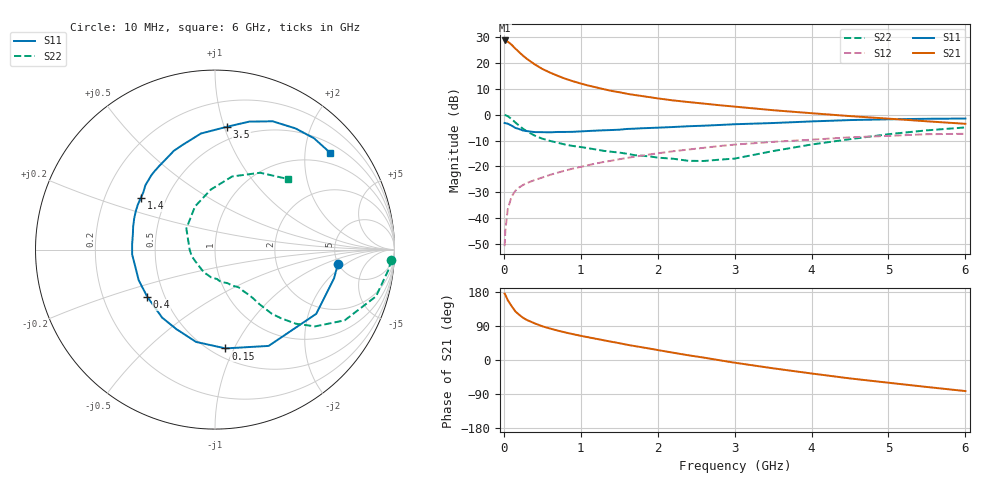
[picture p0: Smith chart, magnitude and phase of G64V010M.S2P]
! SIEMENS Small Signal Semiconductors
! BFG193
! Si NPN RF Bipolar Junction Transistor in SOT223
! VCE = 4 V  IC = 10 mA
! Common Emitter S-Parameters:  August  1996
# GHz  S  MA  R  50
!  f  S11  S21  S12  S22
! GHz  MAG  ANG  MAG  ANG  MAG  ANG  MAG  ANG
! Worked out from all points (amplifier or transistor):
!   36 points, 10 MHz to 6 GHz, reference 50 ohm
!   highest |S21| = 28.6 dB at 10 MHz (marker M1)
!   |S21| within 3 dB of that: start of sweep to 145.5 MHz
!   unconditionally stable (mu >= 1): 884.1 MHz to 2.514 GHz
!   at 250 MHz: K = 0.54, MSG = 24.9 dB, |S12| = -27.2 dB
!   at 1.4 GHz: K = 1.07, MAG = 11.9 dB, |S12| = -17.8 dB
!   at 6 GHz: K = 0.87, MSG = 1.9 dB, |S12| = -7.4 dB
!   S11 on the Smith chart (normalised r, x): 10 MHz: 4.93, -1.53; 150 MHz: 0.58, -0.92; 400 MHz: 0.40, -0.27; 1.4 GHz: 0.36, +0.28; 3.5 GHz: 0.39, +1.02; 6 GHz: 0.71, +2.58
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0.01  0.6889 -6.8  26.88 175.2  0.0029 89.8  0.9842 -3.3
0.02  0.6825 -13.5  26.8 171.8  0.0058 86.3  0.9729 -6.7
0.05  0.6679 -32.4  25.57 158.4  0.0147 75.8  0.9341 -16.2
0.1  0.6142 -60.9  22.3 142.5  0.0262 65.7  0.8232 -28.6
0.15  0.5535 -84.0  18.73 128.3  0.034 57.4  0.7028 -37.5
0.2  0.525 -101.6  15.95 119.2  0.0394 54.1  0.6112 -42.5
0.25  0.4927 -115.8  13.64 111.4  0.0439 51.3  0.5313 -46.1
0.3  0.48 -127.9  11.87 105.5  0.0479 50.8  0.4764 -48.5
0.4  0.4599 -145.1  9.327 96.8  0.0546 50.4  0.3938 -50.8
0.5  0.4581 -158.2  7.597 89.0  0.0611 49.9  0.3434 -52.0
0.6  0.4542 -167.9  6.457 83.1  0.0688 50.5  0.3112 -53.4
0.7  0.4624 -176.6  5.591 77.6  0.0759 51.3  0.286 -55.2
0.9  0.4655 169.4  4.388 68.1  0.0912 50.8  0.2478 -58.0
1.1  0.4827 158.8  3.622 59.9  0.1061 49.7  0.2243 -64.0
1.4  0.5038 145.1  2.861 48.1  0.1291 46.6  0.1918 -73.5
1.7  0.5351 134.1  2.386 36.8  0.1541 42.7  0.1649 -85.7
2.2  0.5757 117.8  1.876 19.3  0.196 34.0  0.1408 -116.3
2.8  0.63 101.5  1.518 -0.5  0.2471 22.3  0.135 -164.6
3.5  0.6874 84.5  1.214 -21.9  0.2979 6.3  0.198 143.7
4.5  0.7837 65.8  0.935 -48.6  0.3644 -13.5  0.3356 93.9
5.5  0.8301 48.4  0.742 -71.2  0.4183 -37.9  0.4965 59.6
6  0.8386 39.9  0.664 -82.0  0.4261 -51.9  0.5653 44.1
